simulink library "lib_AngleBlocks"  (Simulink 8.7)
settings: Solver=ode45  StartTime=0.0  StopTime=10.0  RelTol=1e-3
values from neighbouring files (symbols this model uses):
  Tstep = 0.0005    [TestOrthOscObjO_init.m]    (also in TestWaveMng_init.m = 5e-05)
undefined symbols (not defined in the file or in its folder): defptrAngleabwFB, P_Angleabw_FB, P_TA, set_Angleabw_FB, step_var_to_Angleabw_FB, stepPeriod, T1, Tdelay, u1, u2, u3, work1, y1
libraries: lib_T1Blocks_FB x3, lib_AngleVectorBlocks x2, Lib_FunctionBlocks x1

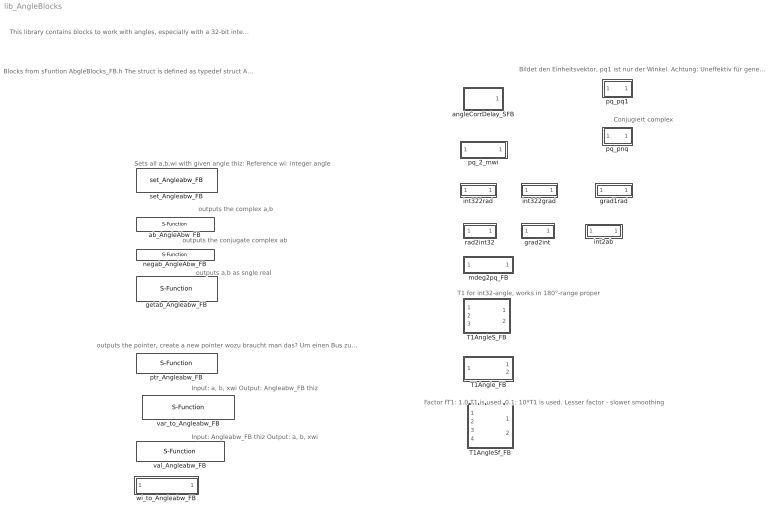
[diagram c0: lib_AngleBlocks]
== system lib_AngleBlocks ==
  note: Conjugiert complex
  note: Bildet den Einheitsvektor, pq1 ist nur der Winkel. Achtung: Uneffektiv für generated code.
  note: Factor fT1: 1.0 T1 is used. 0.1: 10*T1 is used. Lesser factor - slower smoothing
  note: T1 for int32-angle, works in 180°-range proper
  note: Input: a, b, xwi Output: Angleabw_FB thiz
  note: Blocks from sFuntion AbgleBlocks_FB.h The struct is defined as typedef struct Angleabw_FB_t { float a; float b; int32_t wi; } Angleabw_FB; The input left top is a pointer to this struct of type P_Angleabw_FB Such a pointer is returned from otther S-Functions or from the alloc_AngleAbw_FB
  note: outputs the pointer, create a new pointer wozu braucht man das? Um einen Bus zu creieren, ist der var_to_AngleabwFB_CCS richtig. Diese Funktionalität ist auch in S-Function FA enthalten.
  note: outputs a,b as sngle real
  note: outputs the conjugate complex ab
  note: outputs the complex a,b
  note: Sets all a,b,wi with given angle thiz: Reference wi: integer angle
  note: This library contains blocks to work with angles, especially with a 32-bit integer angle representation.
  note: Input: Angleabw_FB thiz Output: a, b, xwi
  T1AngleS_FB : Subsystem
  T1AngleSf_FB : Subsystem
  T1Angle_FB : Subsystem
  ab_AngleAbw_FB : S-Function  FunctionName=ab_AngleAbw_FB  SFunctionDeploymentMode=off  EnableBusSupport=off
  angleCorrDelay_SFB : Subsystem
  getab_Angleabw_FB : S-Function  FunctionName=getab_Angleabw_FB  SFunctionDeploymentMode=off  EnableBusSupport=off
  grad1rad : Subsystem
  grad2int : Subsystem  TreatAsAtomicUnit=on
  int2ab : Subsystem
  int322grad : Subsystem
  int322rad : Subsystem
  mdeg2pq_FB : Subsystem
  negab_AngleAbw_FB : S-Function  FunctionName=negab_AngleAbw_FB  SFunctionDeploymentMode=off  EnableBusSupport=off
  pq_2_mwi : Subsystem  TreatAsAtomicUnit=on
  pq_pnq : Subsystem  TreatAsAtomicUnit=on
  pq_pq1 : Subsystem  TreatAsAtomicUnit=on
  ptr_Angleabw_FB : S-Function  FunctionName=ptr_Angleabw_FB  SFunctionDeploymentMode=off  EnableBusSupport=off
  rad2int32 : Subsystem  TreatAsAtomicUnit=on
  set_Angleabw_FB : Lib_FunctionBlocks/set_Angleabw_FB  SFunctionSpec=set_Angleabw_FB(P_Angleabw_FB u1, int32 u2)  ShowSpec=off
  val_Angleabw_FB : S-Function  FunctionName=AngleabwFB_to_var_CCS  Parameters=SampleTime  SFunctionDeploymentMode=off  EnableBusSupport=off
  var_to_Angleabw_FB : S-Function  LoadFcn=defptrAngleabwFB();  InitFcn=defptrAngleabwFB();  FunctionName=var_to_AngleabwFB_CCS  Parameters=SampleTime  SFunctionDeploymentMode=off  EnableBusSupport=off
  wi_to_Angleabw_FB : Subsystem

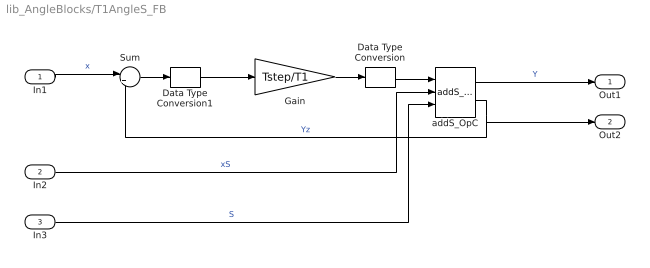
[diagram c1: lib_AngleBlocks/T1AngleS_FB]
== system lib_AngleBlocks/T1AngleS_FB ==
  In1 : Inport  OutDataTypeStr=int32
  In2 : Inport  Port=2  OutDataTypeStr=int32
  In3 : Inport  Port=3  OutDataTypeStr=boolean
  Data Type Conversion : DataTypeConversion  OutDataTypeStr=int32
  Data Type Conversion1 : DataTypeConversion  OutDataTypeStr=single
  Gain : Gain  Gain=Tstep/T1
  Sum : Sum  Inputs=|+-
  addS_OpC : lib_T1Blocks_FB/addS_OpC
  Out1 : Outport  OutDataTypeStr=int32
  Out2 : Outport  Port=2  OutDataTypeStr=int32
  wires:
  Gain/1 -> Data Type Conversion/1
  Sum/1 -> Data Type Conversion1/1
  In1/1 -> Sum/1  "x"
  addS_OpC/1 -> Out1/1  "Y"
  addS_OpC/2 -> Out2/1, Sum/2  "Yz"
  In2/1 -> addS_OpC/2  "xS"
  In3/1 -> addS_OpC/3  "S"
  Data Type Conversion/1 -> addS_OpC/1
  Data Type Conversion1/1 -> Gain/1

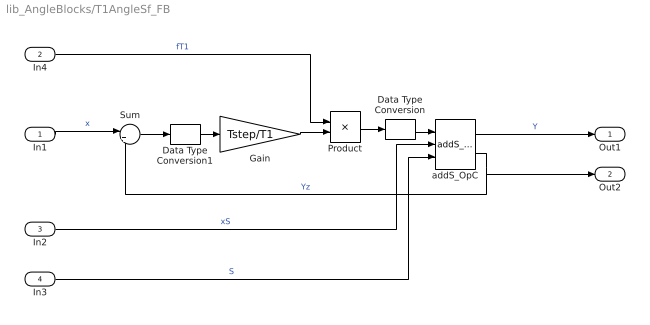
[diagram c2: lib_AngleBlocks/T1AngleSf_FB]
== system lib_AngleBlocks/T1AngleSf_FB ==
  In1 : Inport  OutDataTypeStr=int32
  In4 : Inport  Port=2  OutDataTypeStr=single
  In2 : Inport  Port=3  OutDataTypeStr=int32
  In3 : Inport  Port=4  OutDataTypeStr=boolean
  Data Type Conversion : DataTypeConversion  OutDataTypeStr=int32
  Data Type Conversion1 : DataTypeConversion  OutDataTypeStr=single
  Gain : Gain  Gain=Tstep/T1
  Product : Product
  Sum : Sum  Inputs=|+-
  addS_OpC : lib_T1Blocks_FB/addS_OpC
  Out1 : Outport  OutDataTypeStr=int32
  Out2 : Outport  Port=2  OutDataTypeStr=int32
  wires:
  Data Type Conversion1/1 -> Gain/1
  Data Type Conversion/1 -> addS_OpC/1
  In3/1 -> addS_OpC/3  "S"
  In2/1 -> addS_OpC/2  "xS"
  addS_OpC/2 -> Sum/2, Out2/1  "Yz"
  addS_OpC/1 -> Out1/1  "Y"
  In1/1 -> Sum/1  "x"
  Sum/1 -> Data Type Conversion1/1
  Gain/1 -> Product/2
  Product/1 -> Data Type Conversion/1
  In4/1 -> Product/1  "fT1"

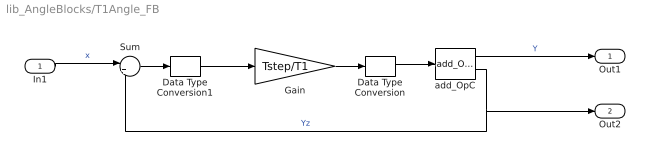
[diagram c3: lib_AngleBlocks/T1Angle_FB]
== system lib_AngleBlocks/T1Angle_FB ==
  In1 : Inport  OutDataTypeStr=int32
  Data Type Conversion : DataTypeConversion  OutDataTypeStr=int32
  Data Type Conversion1 : DataTypeConversion  OutDataTypeStr=single
  Gain : Gain  Gain=Tstep/T1
  Sum : Sum  Inputs=|+-
  add_OpC : lib_T1Blocks_FB/add_OpC  y0=0
  Out1 : Outport  OutDataTypeStr=int32
  Out2 : Outport  Port=2  OutDataTypeStr=int32
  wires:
  Gain/1 -> Data Type Conversion/1
  Sum/1 -> Data Type Conversion1/1
  In1/1 -> Sum/1  "x"
  add_OpC/1 -> Out1/1  "Y"
  add_OpC/2 -> Out2/1, Sum/2  "Yz"
  Data Type Conversion/1 -> add_OpC/1
  Data Type Conversion1/1 -> Gain/1

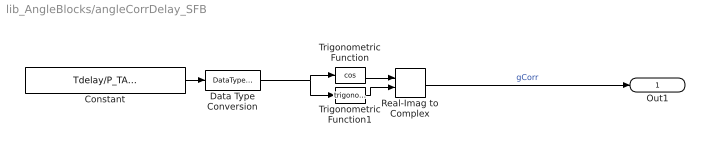
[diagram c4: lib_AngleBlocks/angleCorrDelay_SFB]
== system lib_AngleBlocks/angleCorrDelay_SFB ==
  Constant : Constant  Value=Tdelay/P_TA * 2*pi/stepPeriod
  Data Type Conversion : DataTypeConversion  OutDataTypeStr=single
  Real-Imag to Complex : RealImagToComplex
  Trigonometric Function : Trigonometry  Operator=cos
  Trigonometric Function1 : Trigonometry
  Out1 : Outport
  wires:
  Real-Imag to Complex/1 -> Out1/1  "gCorr"
  Trigonometric Function/1 -> Real-Imag to Complex/1
  Trigonometric Function1/1 -> Real-Imag to Complex/2
  Constant/1 -> Data Type Conversion/1
  Data Type Conversion/1 -> Trigonometric Function/1, Trigonometric Function1/1

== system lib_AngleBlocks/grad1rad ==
  In1 : Inport
  Gain : Gain  Gain=pi/180
  Out1 : Outport
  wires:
  Gain/1 -> Out1/1  "rad"
  In1/1 -> Gain/1  "grad"

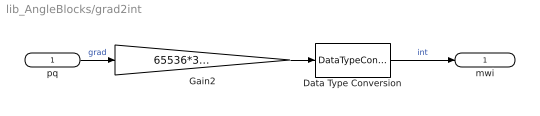
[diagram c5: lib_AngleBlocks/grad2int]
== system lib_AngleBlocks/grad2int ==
  pq : Inport
  Data Type Conversion : DataTypeConversion  OutDataTypeStr=int32  RndMeth=Simplest
  Gain2 : Gain  Gain=65536*32768 / 180
  mwi : Outport  OutDataTypeStr=int32
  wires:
  pq/1 -> Gain2/1  "grad"
  Gain2/1 -> Data Type Conversion/1
  Data Type Conversion/1 -> mwi/1  "int"

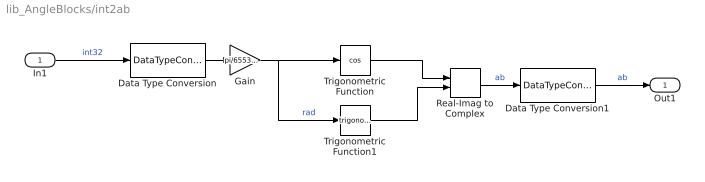
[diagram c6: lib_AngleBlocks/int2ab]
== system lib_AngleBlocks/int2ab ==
  In1 : Inport
  Data Type Conversion : DataTypeConversion  OutDataTypeStr=single
  Data Type Conversion1 : DataTypeConversion  OutDataTypeStr=single
  Gain : Gain  Gain=pi/65536/32768
  Real-Imag to Complex : RealImagToComplex
  Trigonometric Function : Trigonometry  Operator=cos
  Trigonometric Function1 : Trigonometry
  Out1 : Outport  OutDataTypeStr=single
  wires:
  Data Type Conversion/1 -> Gain/1
  Gain/1 -> Trigonometric Function1/1, Trigonometric Function/1  "rad"
  In1/1 -> Data Type Conversion/1  "int32"
  Trigonometric Function/1 -> Real-Imag to Complex/1
  Trigonometric Function1/1 -> Real-Imag to Complex/2
  Real-Imag to Complex/1 -> Data Type Conversion1/1  "ab"
  Data Type Conversion1/1 -> Out1/1  "ab"

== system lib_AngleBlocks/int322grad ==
  In1 : Inport
  Data Type Conversion : DataTypeConversion  OutDataTypeStr=single
  Gain : Gain  Gain=180/65536/32768
  Out1 : Outport
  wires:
  In1/1 -> Data Type Conversion/1  "int32"
  Gain/1 -> Out1/1  "grad"
  Data Type Conversion/1 -> Gain/1

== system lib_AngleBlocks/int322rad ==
  In1 : Inport
  Data Type Conversion : DataTypeConversion  OutDataTypeStr=single
  Gain : Gain  Gain=pi/65536/32768
  Out1 : Outport
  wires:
  Data Type Conversion/1 -> Gain/1
  Gain/1 -> Out1/1  "rad"
  In1/1 -> Data Type Conversion/1  "int32"

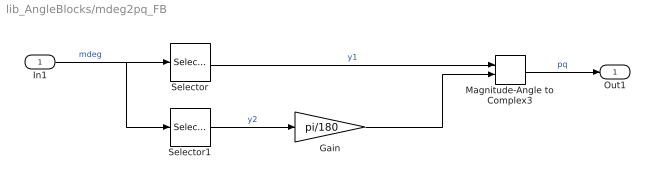
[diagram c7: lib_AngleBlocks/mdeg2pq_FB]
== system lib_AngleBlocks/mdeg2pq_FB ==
  In1 : Inport  PortDimensions=2
  Gain : Gain  Gain=pi/180
  Magnitude-Angle to Complex3 : MagnitudeAngleToComplex
  Selector : Selector  IndexMode=Zero-based  InputPortWidth=2  IndexOptions=Index vector (dialog)  Indices=[0]  OutputSizes=1
  Selector1 : Selector  IndexMode=Zero-based  InputPortWidth=2  IndexOptions=Index vector (dialog)  Indices=[1]  OutputSizes=1
  Out1 : Outport
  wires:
  Gain/1 -> Magnitude-Angle to Complex3/2
  Selector/1 -> Magnitude-Angle to Complex3/1  "y1"
  Magnitude-Angle to Complex3/1 -> Out1/1  "pq"
  In1/1 -> Selector/1, Selector1/1  "mdeg"
  Selector1/1 -> Gain/1  "y2"

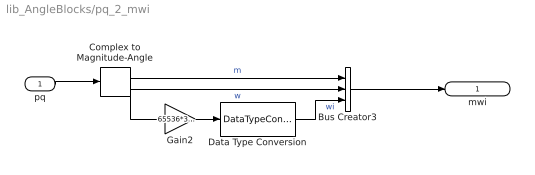
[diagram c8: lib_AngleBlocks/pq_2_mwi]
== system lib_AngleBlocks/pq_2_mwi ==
  pq : Inport
  Bus Creator3 : BusCreator  Inputs='m','w','wi'  OutDataTypeStr=Bus: float_mwi
  Complex to Magnitude-Angle : ComplexToMagnitudeAngle
  Data Type Conversion : DataTypeConversion  OutDataTypeStr=int32  RndMeth=Simplest
  Gain2 : Gain  Gain=65536*32768 / pi
  mwi : Outport
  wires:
  pq/1 -> Complex to Magnitude-Angle/1
  Bus Creator3/1 -> mwi/1
  Complex to Magnitude-Angle/2 -> Bus Creator3/2, Gain2/1  "w"
  Gain2/1 -> Data Type Conversion/1
  Data Type Conversion/1 -> Bus Creator3/3  "wi"
  Complex to Magnitude-Angle/1 -> Bus Creator3/1  "m"

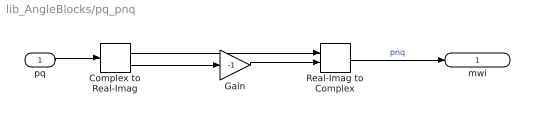
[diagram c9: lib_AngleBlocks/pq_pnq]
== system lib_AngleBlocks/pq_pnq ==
  pq : Inport  OutDataTypeStr=single
  Complex to Real-Imag : ComplexToRealImag
  Gain : Gain  Gain=-1
  Real-Imag to Complex : RealImagToComplex
  mwi : Outport  OutDataTypeStr=single
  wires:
  Real-Imag to Complex/1 -> mwi/1  "pnq"
  Complex to Real-Imag/1 -> Real-Imag to Complex/1
  Complex to Real-Imag/2 -> Gain/1
  pq/1 -> Complex to Real-Imag/1
  Gain/1 -> Real-Imag to Complex/2

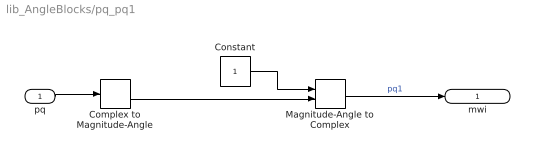
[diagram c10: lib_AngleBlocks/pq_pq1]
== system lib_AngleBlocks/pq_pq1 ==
  pq : Inport  OutDataTypeStr=single
  Complex to Magnitude-Angle : ComplexToMagnitudeAngle
  Constant : Constant  OutDataTypeStr=single
  Magnitude-Angle to Complex : MagnitudeAngleToComplex
  mwi : Outport  OutDataTypeStr=single
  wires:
  pq/1 -> Complex to Magnitude-Angle/1
  Complex to Magnitude-Angle/2 -> Magnitude-Angle to Complex/2
  Constant/1 -> Magnitude-Angle to Complex/1
  Magnitude-Angle to Complex/1 -> mwi/1  "pq1"

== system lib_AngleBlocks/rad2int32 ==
  pq : Inport
  Data Type Conversion : DataTypeConversion  OutDataTypeStr=int32  RndMeth=Simplest
  Gain2 : Gain  Gain=65536*32768 / pi
  mwi : Outport
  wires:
  Data Type Conversion/1 -> mwi/1  "in32"
  Gain2/1 -> Data Type Conversion/1
  pq/1 -> Gain2/1  "rad"

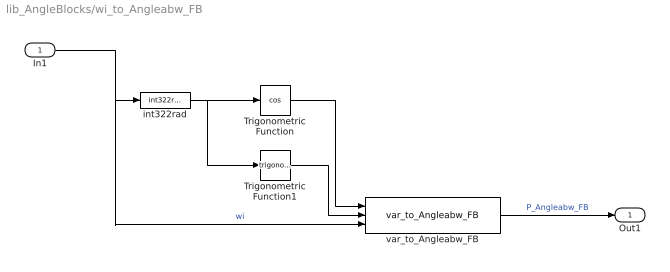
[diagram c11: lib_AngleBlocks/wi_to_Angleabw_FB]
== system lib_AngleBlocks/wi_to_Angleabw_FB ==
  In1 : Inport  OutDataTypeStr=int32  PortDimensions=1
  Trigonometric Function : Trigonometry  Operator=cos
  Trigonometric Function1 : Trigonometry
  int322rad : lib_AngleVectorBlocks/int322rad
  var_to_Angleabw_FB : lib_AngleVectorBlocks/var_to_Angleabw_FB  SFunctionSpec=step_var_to_Angleabw_FB(P_Angleabw_FB work1,single u1, single u2, int32 u3,P_Angleabw_FB y1[1])  SampleTime=-1  ShowSpec=off
  Out1 : Outport  OutDataTypeStr=P_Angleabw_FB
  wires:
  In1/1 -> var_to_Angleabw_FB/3, int322rad/1  "wi"
  int322rad/1 -> Trigonometric Function1/1, Trigonometric Function/1
  Trigonometric Function/1 -> var_to_Angleabw_FB/1
  Trigonometric Function1/1 -> var_to_Angleabw_FB/2
  var_to_Angleabw_FB/1 -> Out1/1  "P_Angleabw_FB"
